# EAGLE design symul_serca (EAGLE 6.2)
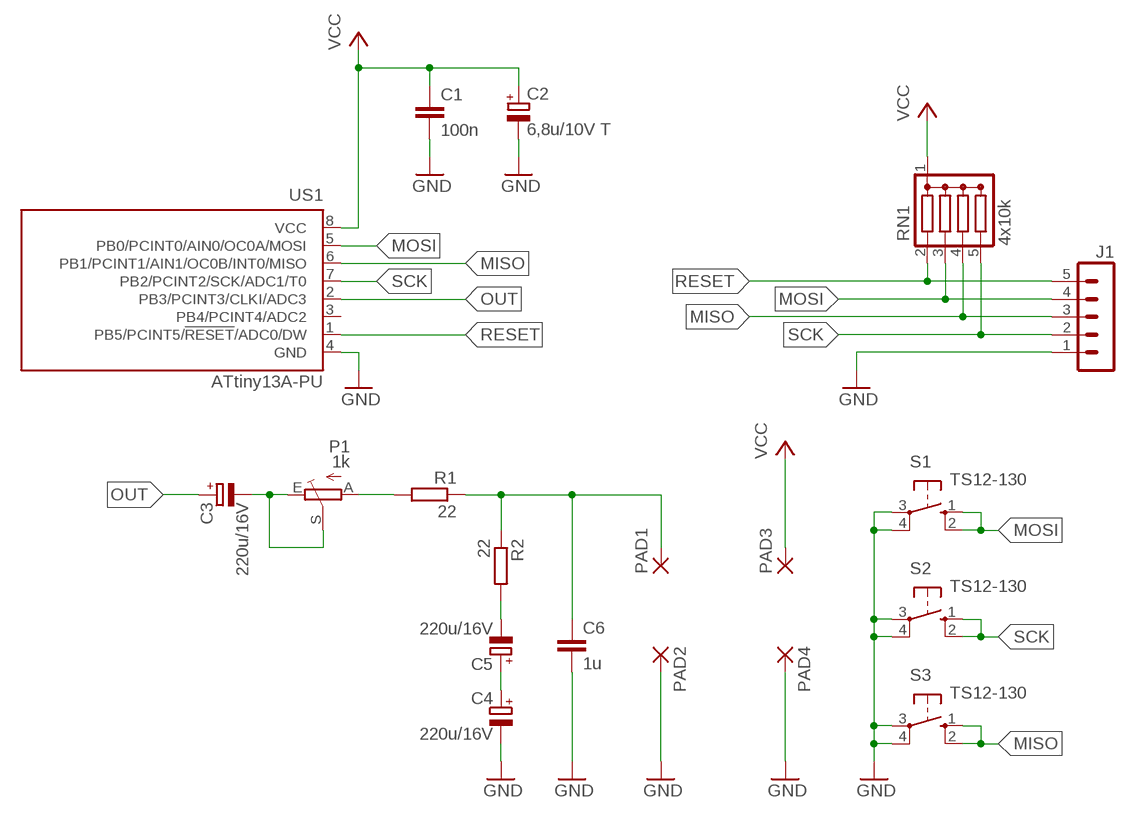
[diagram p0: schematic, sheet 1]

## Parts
C1  100n  C-EU050-025X075  [C050-025X075]
C2  6,8u/10V T  CPOL-EUE2.5-5  [E2,5-5]
C3  220u/16V  CPOL-EUTT2D6L  [TT2D6L]
C4  220u/16V  CPOL-EUTT2D6L  [TT2D6L]
C5  220u/16V  CPOL-EUTT2D6L  [TT2D6L]
C6  1u  C-EU050-025X075  [C050-025X075]
J1  MA05-1  [MA05-1]
P1  1k  TRIM_EU-CA6V  [CA6V]
PAD1  3,81/1,4  [3,81/1,4]
PAD2  3,81/1,4  [3,81/1,4]
PAD3  3,81/1,4  [3,81/1,4]
PAD4  3,81/1,4  [3,81/1,4]
R1  22  R-EU_0207/7  [0207/7]
R2  22  R-EU_0207/7  [0207/7]
RN1  4x10k  DRAB_REZ_1X4  [RN-5]
S1  TS12-130  40-XX  [B3F-40XX]
S2  TS12-130  40-XX  [B3F-40XX]
S3  TS12-130  40-XX  [B3F-40XX]
US1  ATtiny13A-PU  TINY13-20PU  [DIL08]

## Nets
GND: C1.2 C2.- C4.- C6.2 J1.1 PAD2.1(P) PAD4.1(P) S1.3(P) S1.4(P1) S2.3(P) S2.4(P1) S3.3(P) S3.4(P1) US1.4(GND)
MISO: J1.3 RN1.4 S3.1(S) S3.2(S1) US1.6(PB1/PCINT1/AIN1/OC0B/INT0/MISO)
MOSI: J1.4 RN1.3 S1.1(S) S1.2(S1) US1.5(PB0/PCINT0/AIN0/OC0A/MOSI)
N$2: C3.- P1.E P1.S
N$3: C4.+ C5.+
N$4: P1.A R1.2
N$5: C5.- R2.2
N$6: C6.1 PAD1.1(P) R1.1 R2.1
OUT: C3.+ US1.2(PB3/PCINT3/CLKI/ADC3)
RESET: J1.5 RN1.2 US1.1(PB5/PCINT5/!RESET!/ADC0/DW)
SCK: J1.2 RN1.5 S2.1(S) S2.2(S1) US1.7(PB2/PCINT2/SCK/ADC1/T0)
VCC: C1.1 C2.+ PAD3.1(P) RN1.1(C) US1.8(VCC)
Unconnected: US1.3(PB4/PCINT4/ADC2)

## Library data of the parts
C1 C6 = rcl:C-EU: CAPACITOR, European symbol
C2-C5 = rcl:CPOL-EU: POLARIZED CAPACITOR, European symbol
J1 = zlacza_futrzak:MA05-1: PIN HEADER; OC_FARNELL: unknown; OC_NEWARK: unknown
P1 = pot:TRIM_EU-: POTENTIOMETER
PAD1-PAD4 = wirepad:3,81/1,4: THROUGH-HOLE PAD
R1 R2 = rcl:R-EU_: RESISTOR, European symbol
RN1 = inne_futrzak:DRAB_REZ_1X4
S1-S3 = switch-omron:40-XX: OMRON SWITCH; MF: OMRON COMPONENTS USA; MPN: B3F-4000; OC_FARNELL: 176434; OC_NEWARK: 36K3105
US1 = atmel:TINY13: 8-bit AVR Microcontroller with 1K Bytes In-System Programmable Flash Source: http://www.atmel.com/dyn/resources/prod_documents/2535S.pdf; MPN: ATTINY13-20PU; OC_FARNELL: 9171550; OC_NEWARK: 96K6521

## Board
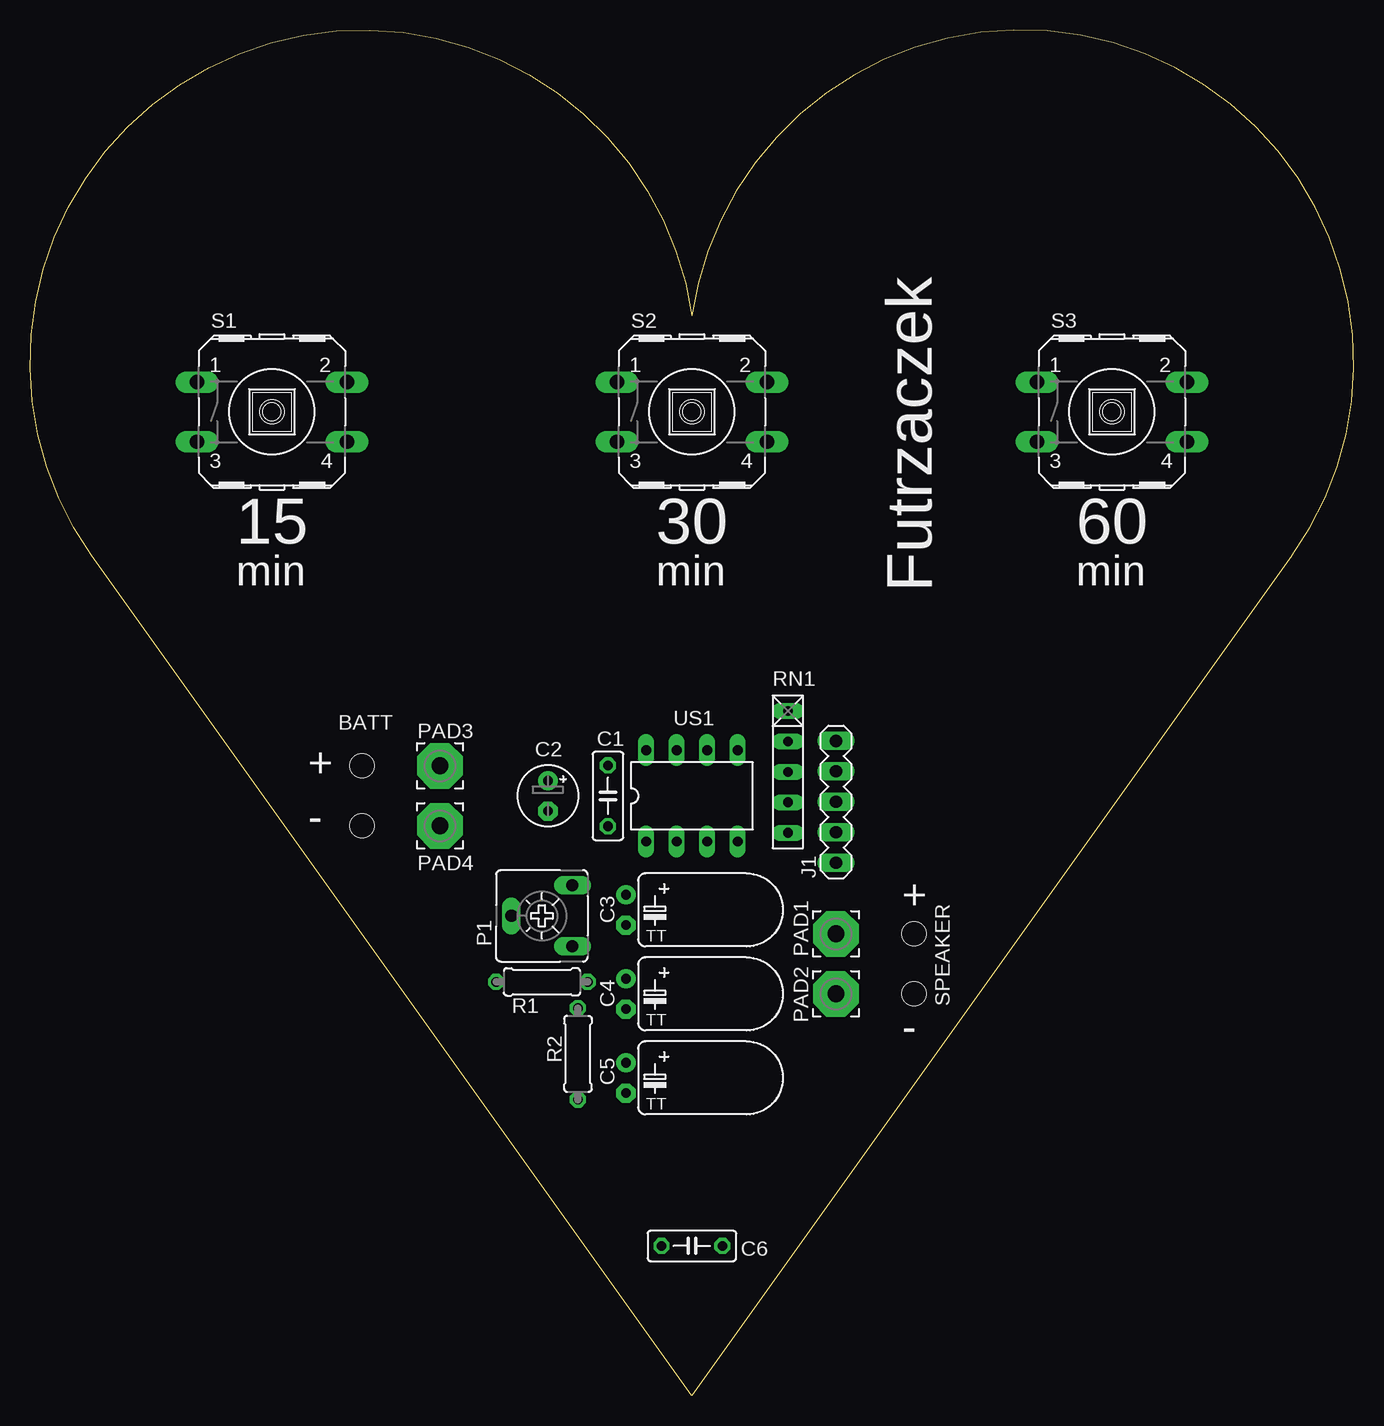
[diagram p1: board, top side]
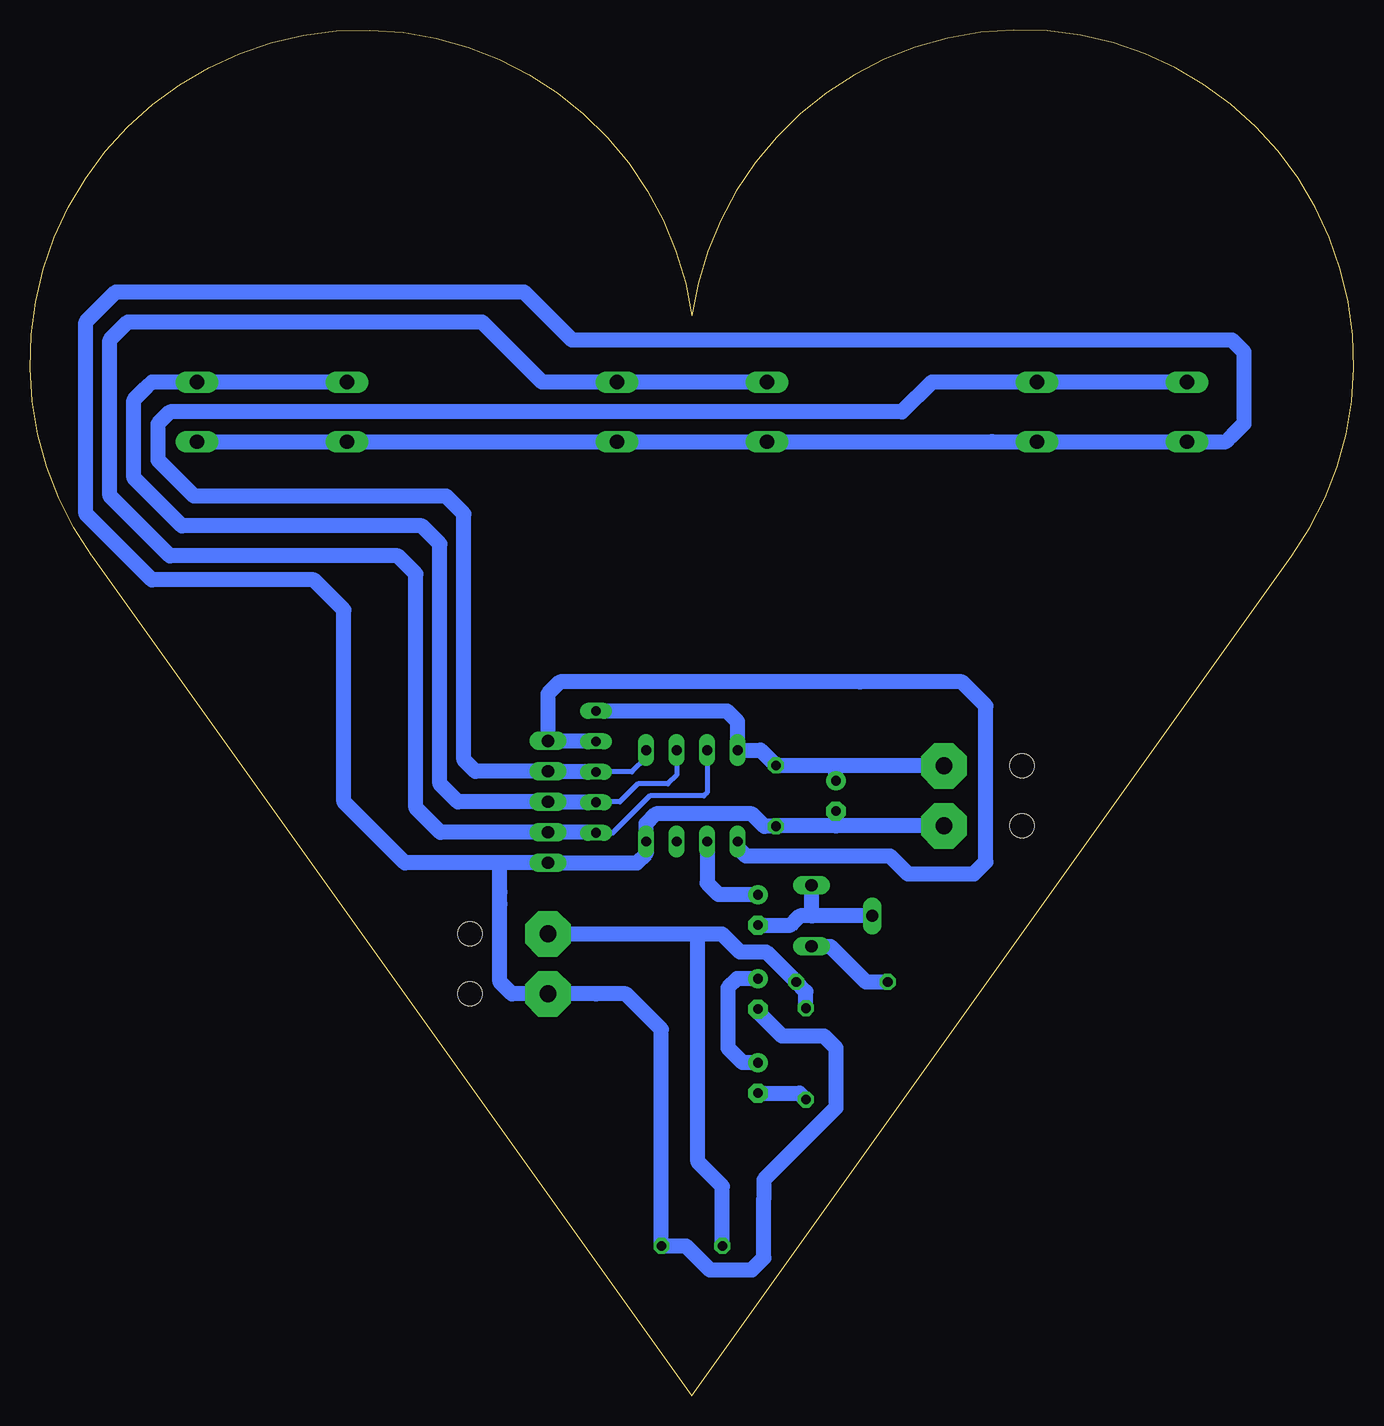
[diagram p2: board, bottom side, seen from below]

Size 110.32 x 113.82 mm. Coordinates in mm from the lower left corner, seen from the top.
Outline: 55.16,0 5.16,70 arc-207 55.16,90 arc-207 105.16,70 55.16,0
Copper layers (1*16): Top 0.035mm / dielectric 1.5mm / Bottom 0.035mm
Design rules: minimum track width 10mil, minimum drill 24mil, track to track 8mil, track to pad 8mil, pad to pad 8mil, via to via 8mil, smd to smd 8mil, copper to edge 15mil, drill to drill 8mil, minimum pad ring 10mil, minimum via ring 8mil, stop-mask expansion 4mil, vias tented up to drill 0mil, thermal gap 10mil
Holes 2 mm at 73.66,33.5 73.66,38.5 27.66,47.5 27.66,52.5

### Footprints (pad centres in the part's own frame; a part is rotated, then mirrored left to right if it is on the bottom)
C050-025X075 = drill 0.813 octagon: 1 -2.54,0; 2 2.54,0
E2,5-5 = drill 0.813 pad 1.6: + -1.27,0 | drill 0.813 pad 1.6 octagon: - 1.27,0
TT2D6L = drill 0.813 pad 1.6: + -1.27,0 | drill 0.813 pad 1.6 octagon: - 1.27,0
MA05-1 = drill 1.016 long: 1 -5.08,0; 2 -2.54,0; 3 0,0; 4 2.54,0; 5 5.08,0
CA6V = drill 1.016 long: A -2.54,-2.54; E 2.54,-2.54; S 0,2.54
3,81/1,4 = drill 1.397 pad 3.81 octagon: 1 0,0
0207/7 = drill 0.813 octagon: 1 -3.81,0; 2 3.81,0
RN-5 = drill 0.813 long: 1 -5.08,0; 2 -2.54,0; 3 0,0; 4 2.54,0; 5 5.08,0
B3F-40XX = drill 1.194 long: 1 -6.248,2.489; 2 6.248,2.489; 3 -6.248,-2.489; 4 6.248,-2.489
DIL08 = drill 0.813 long: 1 -3.81,-3.81; 2 -1.27,-3.81; 3 1.27,-3.81; 4 3.81,-3.81; 5 3.81,3.81; 6 1.27,3.81; 7 -1.27,3.81; 8 -3.81,3.81

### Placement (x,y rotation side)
C1  48.16,50 270 top
C2  43.16,50 270 top
C3  49.66,40.5 270 top
C4  49.66,33.5 270 top
C5  49.66,26.5 270 top
C6  55.16,12.5 0 top
J1  67.16,49.5 90 top
P1  42.66,40 90 top
PAD1  67.16,38.5 0 top
PAD2  67.16,33.5 0 top
PAD3  34.16,52.5 0 top
PAD4  34.16,47.5 0 top
R1  42.66,34.5 180 top
R2  45.66,28.5 270 top
RN1  63.16,52 270 top
S1  20.16,82 0 top
S2  55.16,82 0 top
S3  90.16,82 0 top
US1  55.16,50 0 top

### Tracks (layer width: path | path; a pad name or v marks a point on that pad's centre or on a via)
GND
  Bottom 1.27: 43.16,47.5 48.12,47.5 C1.2 49.12,47.46 50.16,48.5 58.16,48.5 58.97,47.69 US1.4 58.97,45.19 59.74,44.42 J1.1 71.16,44.42 | C2.- 43.16,47.5 | S3.4 S3.3 S2.4 S2.3 30.16,79.51 S1.4 S1.3 10.65,79.51 10.16,80 9.16,81 9.16,87 10.16,88 65.16,88 69.16,92 103.16,92 105.66,89.5 105.66,73.5 100.16,68 86.66,68 86.16,67.5 84.16,65.5 84.16,49.5 79.08,44.42 71.16,44.42 | 43.16,47.5 PAD4.1 33.66,47.5 34.16,47 | C4.- 49.66,32 47.66,30 44.16,30 43.16,29 43.16,24 49.16,18 49.16,16.5 49.16,11.5 50.16,10.5 53.66,10.5 55.66,12.5 C6.2 57.7,30.54 60.66,33.5 63.16,33.5 PAD2.1 70.16,33.5 71.16,34.5 71.16,41 71.16,42 71.16,44.42
MISO
  Bottom 0.406: US1.6 56.43,51.73 57.16,51 59.66,51 61.16,49.5 63.12,49.5 RN1.4
  Bottom 1.27: RN1.4 63.2,49.5 J1.3 74.66,49.5 76.16,51 76.16,71 77.66,72.5 97.66,72.5 101.66,76.5 101.66,83 100.66,84 100.17,84.49 S3.2 S3.1
MOSI
  Bottom 0.406: US1.5 58.97,53.19 60.16,52 RN1.3
  Bottom 1.27: RN1.3 63.2,52.04 J1.4 73.2,52.04 74.16,53 74.16,73.5 75.66,75 81.66,75 96.66,75 99.66,78 99.66,81 98.66,82 37.66,82 35.17,84.49 S1.2 S1.1
N$2
  Bottom 1.27: P1.S 45.16,40 | 45.16,40 46.16,40 46.66,39.5 46.93,39.23 C3.- | P1.E 45.2,40.04 45.16,40
N$3
  Bottom 1.27: C4.+ 51.39,34.77 52.16,34 52.16,29 51.66,28.5 50.93,27.77 C5.+
N$4
  Bottom 1.27: P1.A 43.62,37.46 40.66,34.5 R1.2
N$5
  Bottom 1.27: C5.- 46.2,25.23 R2.2
N$6
  Bottom 1.27: R2.1 45.66,33.69 R1.1 48.97,37 51.16,37 52.66,38.5 54.66,38.5 | PAD1.1 54.66,38.5 | C6.1 52.62,17.46 54.66,19.5 54.66,38.5
OUT
  Bottom 1.27: US1.2 53.89,42.73 53.16,42 52.93,41.77 C3.+
RESET
  Bottom 1.27: RN1.2 63.2,54.58 J1.5 67.16,58.5 66.16,59.5 41.16,59.5 32.66,59.5 30.66,57.5 30.66,44.5 31.66,43.5 37.16,43.5 38.66,45 39.16,45 50.66,45 51.35,45.69 US1.1
SCK
  Bottom 0.406: US1.7 53.89,50.27 54.16,50 58.66,50 61.66,47 61.74,46.92 RN1.5
  Bottom 1.27: RN1.5 63.2,46.96 J1.2 76.12,46.96 78.16,49 78.16,68.5 79.66,70 98.66,70 103.66,75 103.66,88 102.16,89.5 72.66,89.5 68.16,85 67.65,84.49 S2.2 S2.1
VCC
  Bottom 1.27: PAD3.1 43.16,52.5 | 43.16,52.5 48.12,52.5 C1.1 49.43,53.81 US1.8 51.35,56.19 51.66,56.5 52.24,57.08 RN1.1 | C2.+ 43.16,52.5

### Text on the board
tPlace: 15 | 30 | 60 | min | min | min | Futrzaczek | BATT | + | - | + | SPEAKER | -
